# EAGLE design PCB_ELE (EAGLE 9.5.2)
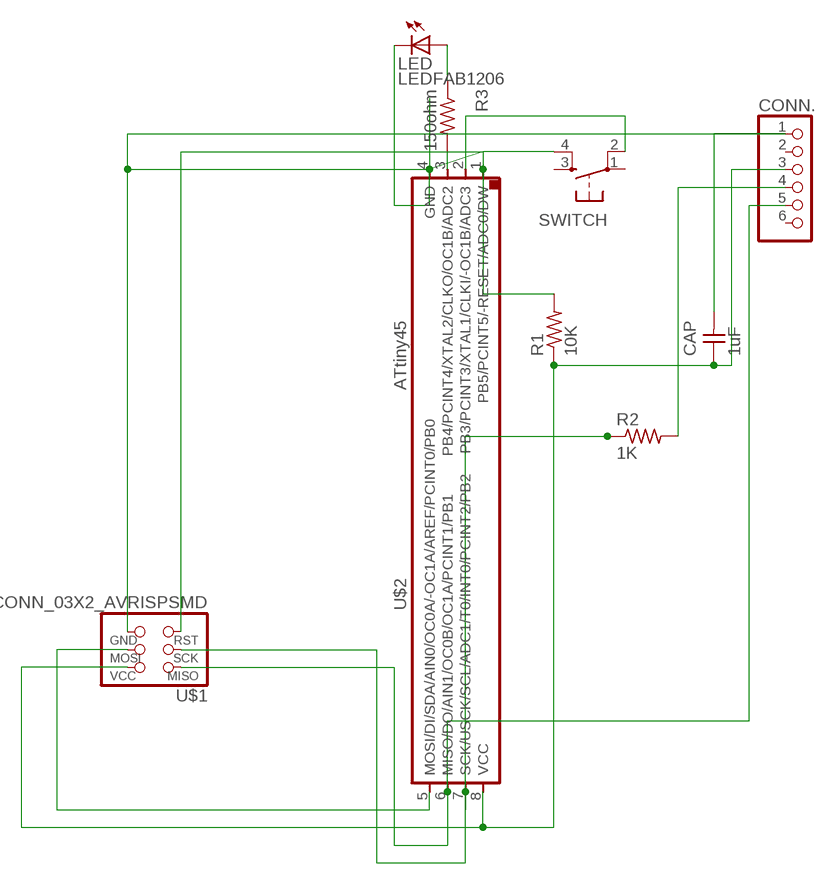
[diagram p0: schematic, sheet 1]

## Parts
CAP  1uF  CAP_UNPOLARIZEDFAB  [C1206FAB]
CONN.  PINHD-1X6  [1X06]
LED  LEDFAB1206  [LED1206FAB]
R1  10K  R1206FAB  [R1206FAB]
R2  1K  R1206FAB  [R1206FAB]
R3  150ohm  R1206FAB  [R1206FAB]
SWITCH  SW_SWITCH_TACTILE_6MM6MM_SWITCH  [6MM_SWITCH]
U$1  CONN_03X2_AVRISPSMD  [2X03SMD]
U$2  UC_ATTINY45SI  [SOIC8]

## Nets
N$1: CAP.2 CONN..1 LED.2(C) SWITCH.4(S1) U$1.6(GND) U$2.4(GND)
N$2: U$1.4(MOSI) U$2.5(MOSI/DI/SDA/AIN0/OC0A/-OC1A/AREF/PCINT0/PB0)
N$3: CAP.1 CONN..3 R1.1 U$1.2(VCC) U$2.8(VCC)
N$4: CONN..4 R2.2
N$6: R1.2 U$1.5(RST) U$2.1(PB5/PCINT5/-RESET/ADC0/DW)
N$7: CONN..5 U$1.1(MISO) U$2.6(MISO/DO/AIN1/OC0B/OC1A/PCINT1/PB1)
N$8: R2.1 U$1.3(SCK) U$2.7(SCK/USCK/SCL/ADC1/T0/INT0/PCINT2/PB2)
N$9: R3.2 U$2.3(PB4/PCINT4/XTAL2/CLKO/OC1B/ADC2)
N$10: LED.1(A) R3.1
N$12: SWITCH.2(P1) U$2.2(PB3/PCINT3/XTAL1/CLKI/-OC1B/ADC3)
Unconnected: CONN..2 CONN..6 SWITCH.1(P) SWITCH.3(S)

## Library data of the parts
CAP = fab:CAP_UNPOLARIZED
CONN. = pinhead:PINHD-1X6: PIN HEADER
LED = fab:LED: LED
R1-R3 = fab:R: Resistor (US Symbol)
SWITCH = fab:SW_SWITCH_TACTILE_6MM: OMRON SWITCH
U$1 = fab:CONN_03X2_AVRISP
U$2 = fab:UC_ATTINY45

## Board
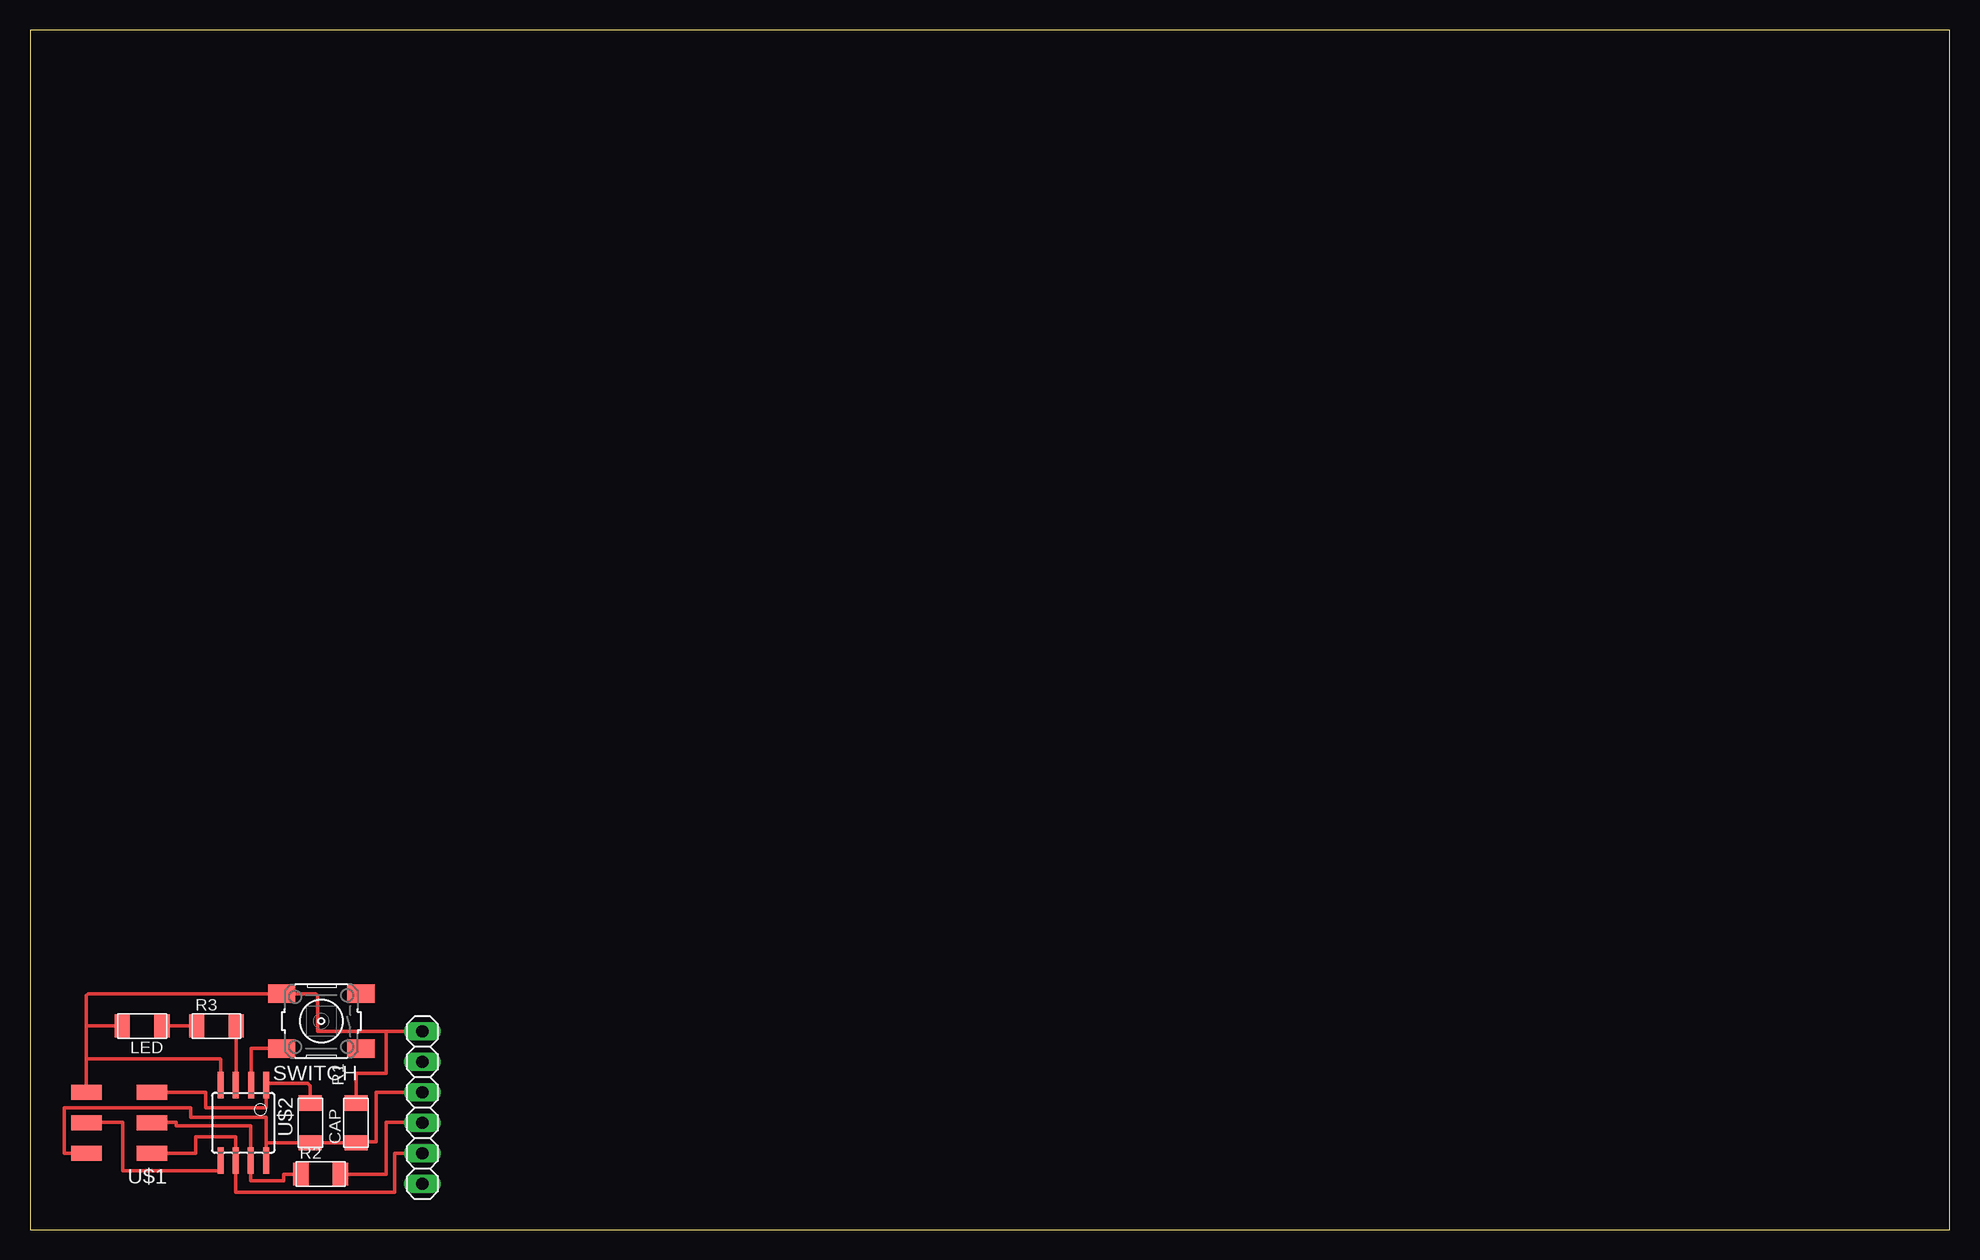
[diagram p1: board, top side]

Size 160 x 100 mm. Coordinates in mm from the lower left corner, seen from the top.
Outline: 0,0 160,0 160,100 0,100 0,0
Copper layers (1*16): Top 0.035mm / dielectric 1.5mm / Bottom 0.035mm
Design rules "default *": minimum track width 12mil, minimum drill 32mil, track to track 16mil, track to pad 16mil, pad to pad 16mil, via to via 16mil, smd to smd 16mil, copper to edge 16mil, drill to drill 16mil, minimum pad ring 10mil, minimum via ring 8mil, stop-mask expansion 4mil, vias tented up to drill 0mil, thermal gap 10mil

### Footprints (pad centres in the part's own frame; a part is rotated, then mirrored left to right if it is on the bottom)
C1206FAB = smd 1.27 x 1.905: 1 -1.651,0; 2 1.651,0
1X06 = drill 1.016 long: 1 -6.35,0; 2 -3.81,0; 3 -1.27,0; 4 1.27,0; 5 3.81,0; 6 6.35,0
LED1206FAB = smd 1.27 x 1.905: 1 -1.651,0; 2 1.651,0
R1206FAB = smd 1.27 x 1.905: 1 -1.651,0; 2 1.651,0
6MM_SWITCH = smd 2.286 x 1.524: 1 -3.302,2.286; 2 3.302,2.286; 3 -3.302,-2.286; 4 3.302,-2.286
2X03SMD = smd 2.54 x 1.27: 1 -2.54,2.54; 2 2.92,2.54; 3 -2.54,0; 4 2.92,0; 5 -2.54,-2.54; 6 2.92,-2.54
SOIC8 = smd 0.5 x 2.2: 1 -1.905,-3.154; 2 -0.645,-3.154; 3 0.625,-3.154; 4 1.895,-3.154; 5 1.905,3.154; 6 0.635,3.154; 7 -0.635,3.154; 8 -1.905,3.154

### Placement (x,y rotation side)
CAP  27.18,8.89 90 top
CONN.  32.72,10.16 270 top
LED  9.35,16.97 180 top
R1  23.37,8.89 90 top
R2  24.23,4.62 0 top
R3  15.54,16.97 0 top
SWITCH  24.28,17.37 180 top
U$1  7.62,8.89 180 top
U$2  17.78,8.89 180 top

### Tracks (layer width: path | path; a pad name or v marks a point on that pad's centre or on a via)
N$1
  Top 0.305: U$1.6 4.7,14.22 | 15.85,12.04 U$2.4 15.88,14.19 15.85,14.22 4.7,14.22 | 4.7,14.22 4.7,16.97 | 4.7,16.97 4.7,19.51 4.85,19.66 SWITCH.4 23.82,19.66 23.98,19.51 23.98,16.51 29.67,16.51 | LED.2 4.7,16.97 | 29.67,16.51 CONN..1 | CAP.2 27.18,13.01 29.67,13.01 29.67,16.51
N$2
  Top 0.305: U$1.4 4.7,8.94 7.72,8.94 7.72,4.88 15.88,4.88 U$2.5
N$3
  Top 0.305: U$1.2 2.85,6.35 2.85,10.16 13.41,10.16 13.41,9.35 19.68,9.35 U$2.8 19.68,7.24 R1.1 CAP.1 27.18,7.32 28.85,7.32 28.85,11.43 CONN..3
N$4  (via drill 0.81)
  Top 0.305: R2.2 29.67,4.62 29.67,8.94 32.66,8.94 CONN..4
  other vias: 32.72,8.89
N$6
  Top 0.305: U$1.5 14.63,11.43 14.63,10.16 19.68,10.16 U$2.1 19.83,12.19 23.16,12.19 23.37,11.99 R1.2 23.57,10.54
N$7
  Top 0.305: U$1.1 13.82,6.35 13.82,7.72 17.14,7.72 U$2.6 17.14,3.11 30.38,3.11 30.38,6.35 CONN..5
N$8
  Top 0.305: U$1.3 10.16,8.94 12.19,8.94 12.19,8.64 18.41,8.64 U$2.7 18.41,4.06 21.13,4.06 21.13,4.62 R2.1
N$9
  Top 0.305: R3.2 17.2,12.6 17.07,12.6 17.07,12.04 U$2.3
N$10
  Top 0.305: R3.1 LED.1
N$12
  Top 0.305: U$2.2 18.43,15.09 SWITCH.2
